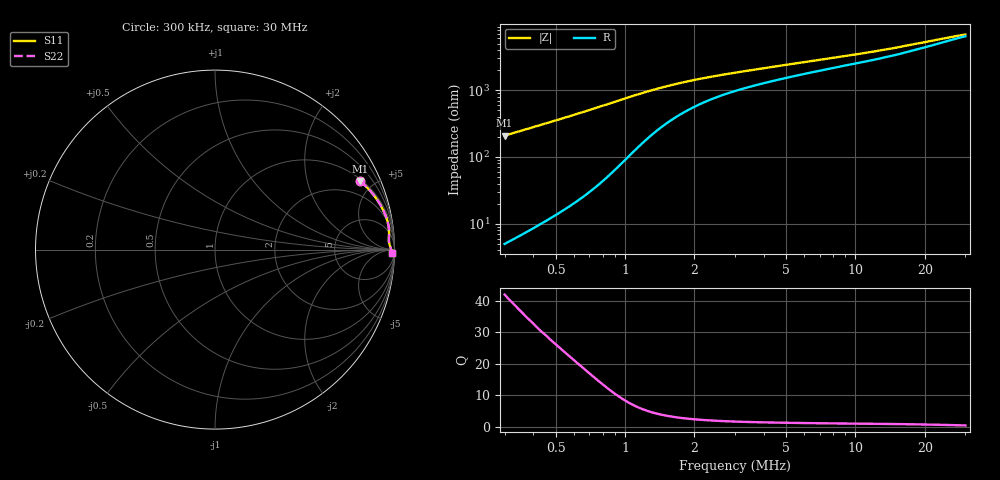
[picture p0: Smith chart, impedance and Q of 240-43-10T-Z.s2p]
! ListType=Log
!!FT240-43 10T Balun Z Measurement S21 Through
# MHZ S RI R 50
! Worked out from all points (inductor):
!   101 points, 300 kHz to 30 MHz, reference 50 ohm
!   read as one part in series: L = 111 uH near 300 kHz
!   highest Q = 42 at 300 kHz (marker M1), where L = 111 uH
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0.3  0.8079 0.3818  0.1919 -0.3822  0.1919 -0.3822  0.8079 0.3818
0.3444461  0.8458 0.3474  0.1539 -0.3479  0.1539 -0.348  0.8458 0.3475
0.395477  0.8771 0.3129  0.1226 -0.3134  0.1226 -0.3134  0.8771 0.3129
0.4540684  0.9024 0.2792  0.0973 -0.2798  0.0973 -0.2797  0.9024 0.2792
0.5213402  0.9226 0.2471  0.0771 -0.2477  0.0771 -0.2477  0.9227 0.2471
0.7196499  0.9539 0.1802  0.0459 -0.1809  0.0459 -0.1809  0.9539 0.1801
0.9486833  0.9666 0.1327  0.0331 -0.1336  0.0331 -0.1336  0.9666 0.1326
1.140568  0.9694 0.1071  0.0302 -0.1081  0.0302 -0.1081  0.9694 0.1071
1.309548  0.9698 0.0914  0.0299 -0.0926  0.0299 -0.0927  0.9699 0.0915
1.503562  0.9695 0.0787  0.0301 -0.08  0.0301 -0.08  0.9696 0.0787
1.72632  0.9693 0.0681  0.0305 -0.0697  0.0305 -0.0698  0.9692 0.0681
1.98208  0.9689 0.0595  0.0308 -0.0613  0.0308 -0.0613  0.9689 0.0595
2.275733  0.9689 0.0523  0.0308 -0.0544  0.0308 -0.0544  0.9689 0.0523
3  0.9696 0.041  0.0301 -0.0437  0.0301 -0.0437  0.9696 0.0411
4.141153  0.9716 0.031  0.0281 -0.0348  0.0281 -0.0348  0.9716 0.031
5.459103  0.9737 0.0238  0.026 -0.0288  0.026 -0.0288  0.9738 0.0238
7.535659  0.9762 0.0164  0.0233 -0.0232  0.0233 -0.0232  0.9763 0.0164
10.40211  0.9788 0.00918  0.0207 -0.0187  0.0207 -0.0187  0.9788 0.00916
15.74422  0.9815 -0.000811  0.0173 -0.0135  0.0172 -0.0135  0.9815 -0.000778
20.75493  0.9828 -0.0083  0.0153 -0.00991  0.0153 -0.00991  0.9829 -0.00832
26.12891  0.984 -0.0156  0.0141 -0.00695  0.0141 -0.00696  0.984 -0.0155
30  0.9841 -0.0205  0.0135 -0.00511  0.0135 -0.00511  0.9842 -0.0205
